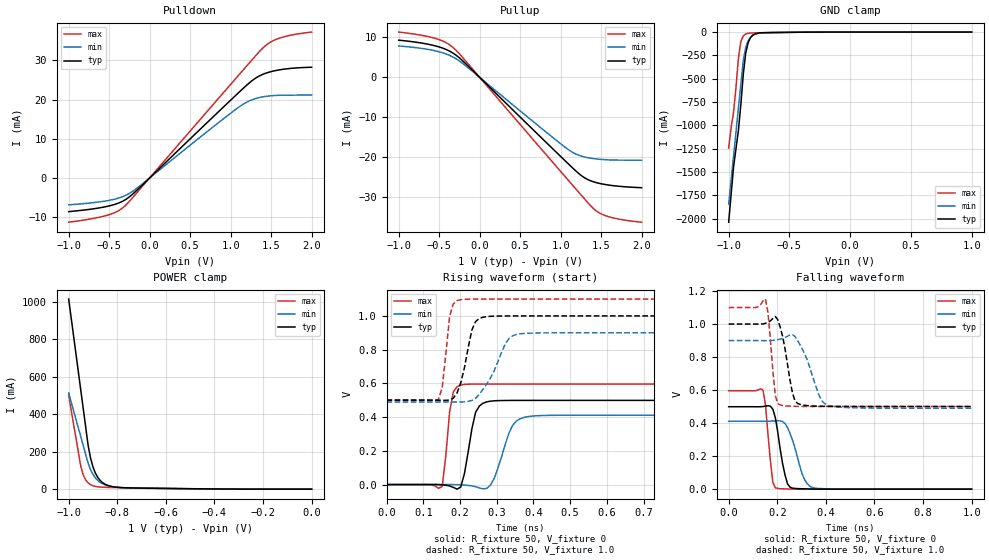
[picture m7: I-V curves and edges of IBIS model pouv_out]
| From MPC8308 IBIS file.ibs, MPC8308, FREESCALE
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[Model]   pouv_out
Model_type 3-state
Enable Active-High
Polarity Non-Inverting
Vmeas=0.5
C_comp   857fF   831fF   883fF
[Temperature Range] 65   125   -40
[Voltage Range]   1.0   0.9   1.1
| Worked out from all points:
|   slope of the pulldown table from 0 to 0.15 V, typ, clamps not added: 50 ohm
|   slope of the pullup table from 0 to 0.15 V, typ, clamps not added: 50 ohm
|   GND clamp passes 1 mA (typ) near -0.36 V on its own axis
|   POWER clamp passes 1 mA (typ) near -0.38 V on its own axis
|   falling waveform, R_fixture 50, V_fixture 0: 20-80 % time 34.1ps typ, 50.7ps min, 22.3ps max; typ from 0.499 V to 0 V
|   falling waveform, R_fixture 50, V_fixture 1.0: 20-80 % time 34.8ps typ, 58ps min, 21.1ps max; typ from 1 V to 0.501 V
|   rising waveform, R_fixture 50, V_fixture 0: 20-80 % time 24.6ps typ, 37.7ps min, 17ps max; typ from 0 V to 0.499 V
|   rising waveform, R_fixture 50, V_fixture 1.0: 20-80 % time 29.2ps typ, 55ps min, 17.1ps max; typ from 0.501 V to 1 V
[Pullup]
-1V       9.32mA     7.87mA     11.35mA
-580mV    8.054mA    6.783mA    9.944mA
-450mV    7.278mA    6.108mA    9.045mA
-360mV    6.449mA    5.398mA    7.994mA
-180mV    3.58mA     3.017mA    4.268mA
1.09V     -21.61mA   -18.06mA   -25.71mA
1.18V     -23.34mA   -19.16mA   -27.82mA
1.27V     -24.86mA   -19.85mA   -29.93mA
1.39V     -26.11mA   -20.35mA   -32.63mA
1.48V     -26.62mA   -20.56mA   -34.04mA
1.58V     -26.99mA   -20.7mA    -34.89mA
2V        -27.69mA   -20.81mA   -36.35mA
[Pulldown]
-1V       -8.604mA   -6.862mA   -11.3mA
-550mV    -7.37mA    -5.9mA     -9.672mA
-420mV    -6.681mA   -5.355mA   -8.745mA
-330mV    -5.912mA   -4.76mA    -7.601mA
-240mV    -4.669mA   -3.824mA   -5.731mA
-150mV    -2.993mA   -2.499mA   -3.592mA
1.09V     21.61mA    17.92mA    26.02mA
1.27V     24.92mA    20.01mA    30.29mA
1.42V     26.64mA    20.78mA    33.58mA
1.52V     27.26mA    21.02mA    34.99mA
1.64V     27.72mA    21.11mA    35.93mA
2V        28.26mA    21.19mA    37.24mA
[GND Clamp]
-1V       -2.039A    -1.845A    -1.243A
-980mV    -1.743A    -1.588A    -1.027A
-960mV    -1.448A    -1.331A    -861.2mA
-940mV    -1.252A    -1.075A    -596.4mA
-920mV    -1.057A    -818.1mA   -280.9mA
-900mV    -781.5mA   -561.4mA   -103.4mA
-880mV    -456mA     -304.7mA   -42.05mA
-860mV    -228.1mA   -166.9mA   -20.69mA
-840mV    -113.8mA   -92.92mA   -13.07mA
-800mV    -32.13mA   -31.58mA   -8.914mA
-620mV    -4.646mA   -4.49mA    -4.844mA
1V        410.4nA    7.402uA    123.8nA
[POWER Clamp]
-1V       1.014A     513.2mA    500.1mA
-950mV    526.8mA    279.3mA    120.9mA
-940mV    429.3mA    232.5mA    75.94mA
-930mV    331.9mA    185.7mA    49.26mA
-920mV    234.4mA    138.9mA    33.39mA
-910mV    166.3mA    104.4mA    23.92mA
-900mV    118.7mA    78.91mA    18.22mA
-880mV    62.11mA    46.13mA    12.63mA
-860mV    34.35mA    28.17mA    10.4mA
-820mV    13.77mA    12.73mA    8.711mA
-760mV    7.252mA    6.614mA    7.358mA
0V        410.4nA    144.6nA    131.1nA
[Falling Waveform]
R_fixture=50
V_fixture=0
V_fixture_min=0
V_fixture_max=0
0s        499.3mV    411.4mV    596.2mV
141.4ps   500.4mV    411.2mV    599.7mV
151.5ps   503.1mV    411.3mV    510.8mV
181.8ps   484.8mV    412.6mV    41.2mV
191.9ps   433.7mV    413.6mV    8.419mV
232.3ps   83.75mV    396.7mV    1.591mV
262.6ps   6.25mV     297.2mV    584.4uV
313.1ps   1.797mV    56.86mV    89.23uV
353.5ps   753.7uV    6.227mV    20.52uV
1ns       1.739uV    3.818uV    2.896uV
[Falling Waveform]
R_fixture=50
V_fixture=1.0
V_fixture_min=0.9
V_fixture_max=1.1
0s        1V         900mV      1.1V
151.5ps   1.005V     899.6mV    1.151V
161.6ps   1.011V     899.6mV    1.071V
191.9ps   1.046V     902.5mV    567.2mV
212.1ps   981mV      908.5mV    510.2mV
262.6ps   582mV      935.8mV    502.1mV
282.8ps   519.9mV    902.9mV    501.4mV
373.7ps   502.2mV    563.3mV    500.8mV
404ps     501.4mV    511.2mV    500.8mV
1ns       500.6mV    490.1mV    500.8mV
[Rising Waveform]
R_fixture=50
V_fixture=0
V_fixture_min=0
V_fixture_max=0
0s        1.736uV    3.698uV    2.896uV
151.5ps   -1.524mV   243.6uV    -11.36mV
171.7ps   -7.963mV   169.5uV    431.2mV
181.8ps   -16.5mV    -157uV     550.5mV
202ps     -14.52mV   -1.704mV   590.5mV
242.4ps   428.3mV    -12.81mV   596mV
272.7ps   490.5mV    -22.4mV    596.2mV
343.4ps   499.1mV    351.9mV    596.2mV
373.7ps   499.2mV    397.9mV    596.2mV
1ns       499.2mV    411.4mV    596.2mV
[Rising Waveform]
R_fixture=50
V_fixture=1.0
V_fixture_min=0.9
V_fixture_max=1.1
0s        500.6mV    490.1mV    500.8mV
141.4ps   500.2mV    490.2mV    505mV
151.5ps   499.6mV    490.1mV    575.4mV
171.7ps   501.3mV    489.9mV    997.8mV
191.9ps   543.2mV    489.5mV    1.091V
232.3ps   917.1mV    498.8mV    1.1V
262.6ps   992.3mV    564.9mV    1.1V
323.2ps   999.7mV    834.1mV    1.1V
353.5ps   999.9mV    890mV      1.1V
1ns       1V         900mV      1.1V
[Ramp]
R_load=50
dV/dt_r   2.995E-1/2.350E-11   2.468E-1/3.722E-11   3.577E-1/1.492E-11
dV/dt_f   2.996E-1/3.430E-11   2.460E-1/5.769E-11   3.595E-1/1.996E-11
|[End   pouv_out
